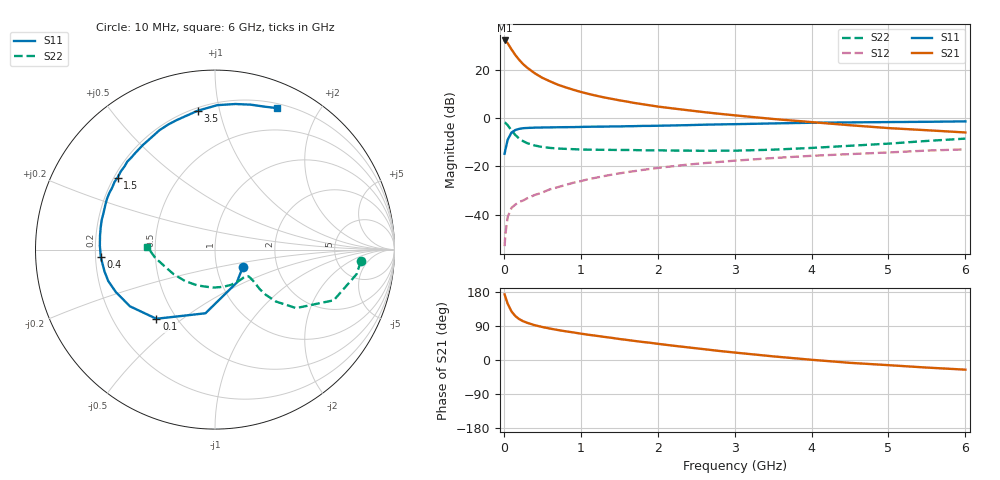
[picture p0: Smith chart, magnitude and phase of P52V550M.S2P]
! SIEMENS Small Signal Semiconductors
! BFP183
! Si NPN RF Bipolar Junction Transistor in SOT143
! VCE = 2.5 V  IC = 50 mA
! Common Emitter S-Parameters:  March  1996
# GHz  S  MA  R  50
!  f  S11  S21  S12  S22
! GHz  MAG  ANG  MAG  ANG  MAG  ANG  MAG  ANG
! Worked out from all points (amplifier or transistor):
!   36 points, 10 MHz to 6 GHz, reference 50 ohm
!   highest |S21| = 32.3 dB at 10 MHz (marker M1)
!   |S21| within 3 dB of that: start of sweep to 85.76 MHz
!   unconditionally stable (mu >= 1): start of sweep to 22.08 MHz; 265.4 MHz to end of sweep
!   at 250 MHz: K = 0.98, MSG = 28.3 dB, |S12| = -34.2 dB
!   at 1.4 GHz: K = 1.48, MAG = 11.7 dB, |S12| = -23.5 dB
!   at 6 GHz: K = 1.13, MAG = 1.3 dB, |S12| = -12.9 dB
!   S11 on the Smith chart (normalised r, x): 10 MHz: 1.34, -0.27; 100 MHz: 0.39, -0.40; 400 MHz: 0.22, -0.03; 1.5 GHz: 0.21, +0.32; 3.5 GHz: 0.22, +0.86; 6 GHz: 0.25, +1.50
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0.01  0.1827 -31.8  41.23 173.1  0.0022 65.6  0.8151 -4.6
0.02  0.2202 -56.6  40.7 166.6  0.0039 67.6  0.801 -9.8
0.05  0.3587 -98.5  36.12 148.4  0.0089 67.0  0.7195 -23.1
0.1  0.5052 -130.3  26.81 128.0  0.0138 53.2  0.5572 -35.8
0.15  0.5695 -146.3  20.48 115.8  0.0161 49.4  0.4467 -40.4
0.2  0.6009 -156.8  16.24 107.9  0.0183 49.9  0.3785 -41.7
0.25  0.62 -163.6  13.33 102.4  0.0195 49.4  0.3343 -41.5
0.3  0.6274 -168.7  11.33 98.4  0.0216 52.2  0.3053 -40.5
0.4  0.6376 -176.1  8.622 91.9  0.0254 54.6  0.2715 -39.2
0.5  0.6419 178.0  6.914 87.1  0.0286 56.0  0.2522 -38.7
0.6  0.6451 173.3  5.839 82.9  0.0334 58.3  0.2419 -38.6
0.7  0.6488 169.0  4.983 79.2  0.0369 60.5  0.235 -39.1
0.9  0.6536 161.9  3.916 72.9  0.0455 60.7  0.2276 -41.3
1.1  0.665 154.8  3.204 66.6  0.0543 60.9  0.2225 -44.6
1.5  0.675 143.5  2.357 55.5  0.0714 59.0  0.2189 -52.9
1.8  0.6922 134.9  1.957 47.7  0.0842 57.4  0.2158 -60.9
2.2  0.7078 124.6  1.595 37.8  0.1008 53.4  0.2129 -72.0
2.8  0.7441 110.5  1.238 23.9  0.1237 47.4  0.2118 -91.5
3.5  0.78 97.0  0.965 9.6  0.1488 40.7  0.2222 -116.0
4.5  0.8191 82.0  0.715 -7.5  0.1797 30.6  0.2678 -149.1
5.5  0.8426 71.0  0.563 -20.0  0.2128 21.6  0.3374 -172.5
6  0.8601 66.4  0.506 -25.5  0.2259 16.5  0.377 177.7
